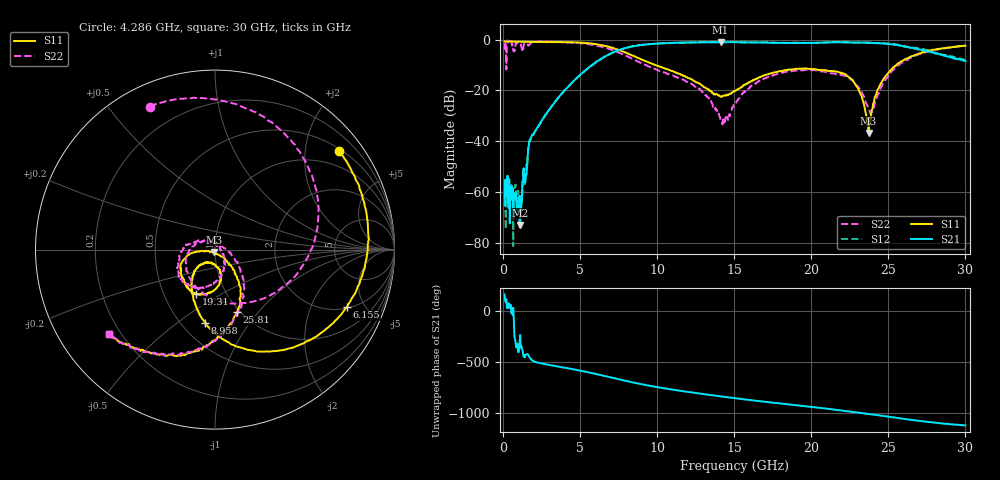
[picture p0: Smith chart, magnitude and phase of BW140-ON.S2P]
!  2-Port S-parameters saved by WinCal
! VAR MeasName=S-Parameters (CALIBRATED_DATA) read from VNA (N5244A)
! VAR MeasDate=11/21/2012 4:48:38 PM
! VAR NAME=128931 2
! VAR FILENAME=128931 2.S2P
! VAR DATE=11/21/2012 4:48:38 PM
! VAR PHYS_PORTS=1,2
# Hz S MA R 50
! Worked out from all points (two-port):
!   801 points, 100 MHz to 30 GHz, reference 50 ohm
!   highest |S21| = -1.01 dB at 14.12 GHz (marker M1); lowest = -72.7 dB at 1.109 GHz (marker M2)
!   |S21| within 3 dB of the highest: 7.576 GHz to 27.09 GHz (19.51 GHz wide, 113 % of centre)
!   lowest |S11| = -36.7 dB at 23.72 GHz (marker M3), VSWR 1.03, Z = 49.5 - j1.35 ohm
!   |S11| at or under -10 dB: 9.878 GHz to 25.51 GHz (15.64 GHz wide, 88.4 % of centre)
!   |S22| runs from -33.3 to -0.4 dB; largest |S21 - S12| = 0.047
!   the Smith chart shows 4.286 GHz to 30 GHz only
!   S11 on the Smith chart (normalised r, x): 4.286 GHz: 0.55, +2.75; 6.155 GHz: 2.09, -3.72; 8.958 GHz: 0.65, -0.64; 19.31 GHz: 0.72, -0.38; 25.81 GHz: 0.97, -0.78; 30 GHz: 0.16, -0.34
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1e8  0.917 176.4  0.000569 164.7  0.001147 150.1  0.6321 78.6
2.86875e8  0.9136 170.2  0.00213 28.7  0.0006072 26.4  0.9583 -82.0
3.99e8  0.9129 166.4  0.001815 36.0  0.0006311 72.4  0.919 -114.2
1.109125e9  0.9057 142.7  0.0002313 126.4  0.0003732 96.2  0.8682 -173.2
1.81925e9  0.8988 119.1  0.01214 -113.8  0.01211 -116.1  0.8649 179.7
4.286e9  0.8829 38.7  0.1246 155.6  0.1232 155.6  0.8757 114.5
5.10825e9  0.8651 11.6  0.216 131.3  0.216 131.4  0.8409 91.8
6.15475e9  0.8014 -23.4  0.3824 97.2  0.3769 97.7  0.7502 58.4
7.388125e9  0.642 -62.3  0.6004 53.9  0.6004 53.9  0.5758 10.4
8.957875e9  0.41 -97.8  0.781 1.5  0.783 1.7  0.3456 -59.1
1.007912e10  0.3008 -113.6  0.8363 -29.8  0.835 -29.7  0.2482 -107.8
1.202262e10  0.1756 -131.9  0.8725 -75.8  0.8678 -75.8  0.1452 -178.8
1.411562e10  0.07639 -109.4  0.8905 -119.0  0.8797 -118.7  0.02567 86.7
1.505e10  0.09909 -81.4  0.884 -136.9  0.8944 -137.1  0.0558 -31.6
1.673188e10  0.1861 -81.9  0.8705 -167.6  0.8799 -167.5  0.1614 -80.1
1.931075e10  0.2672 -113.5  0.8577 148.4  0.8681 147.7  0.2468 -128.8
2.005825e10  0.2615 -124.4  0.8562 135.7  0.8603 135.4  0.2495 -141.5
2.256238e10  0.1706 -164.5  0.8761 89.8  0.8751 89.4  0.1677 174.3
2.3721e10  0.01464 -111.1  0.8659 67.8  0.8715 66.9  0.04187 101.2
2.502912e10  0.2266 -53.7  0.8133 40.0  0.8327 40.6  0.1985 -44.0
2.5814e10  0.3693 -70.6  0.76 22.1  0.7549 22.4  0.3445 -64.4
3e10  0.756 -141.5  0.3759 -45.5  0.3916 -48.0  0.753 -141.4
